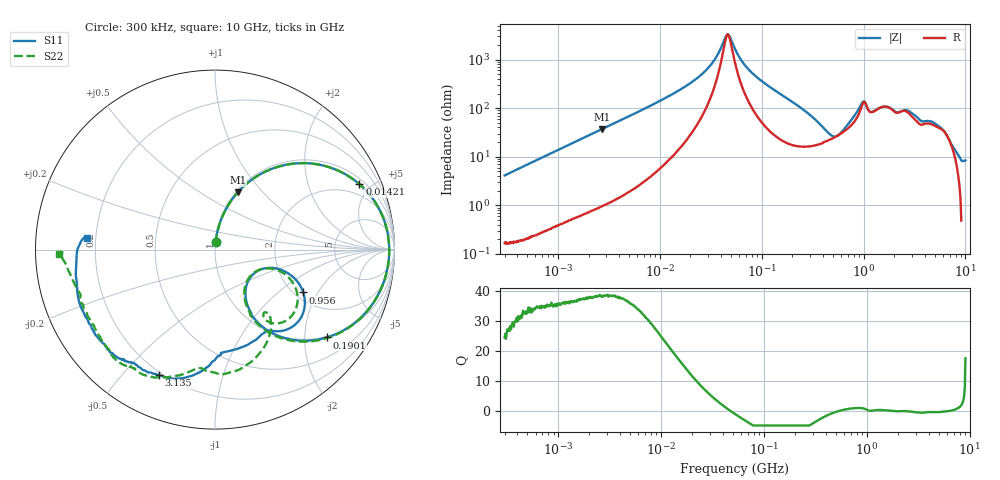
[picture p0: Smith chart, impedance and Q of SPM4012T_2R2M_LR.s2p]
! S-Parameter Data Generated by TDK Corporation
! Copyright(C) 2019 TDK Corporation.
! All Rights Reserved.
! TDK P/N: SPM4012T-2R2M-LR (Inductor)
! Property: L=2.2uH at 100kHz
! Size(LxWxT): 4.4x4.1x1.2mm
! Model Type: s2p (Touchstone File Format Version 1.0)
! Frequency: DC=Yes Start=0.3MHz Stop=10000MHz 802points Log-sweep
! Model Generated on Sep. 23, 2019
! Port Assignments:
!  1 ---@@@--- 2
! Applicable Conditions:
!  Temperature = 25 degC
!  DC Bias Current = 0 A
!  Small Signal Operation
! Terms and conditions regarding TDK Simulation Models
! (1)This simulation model is being provided solely for informational purposes. Please refer to the specifications of the products in terms of detailed characteristics of such products.
! (2)In no event shall TDK Corporation of any of its subsidiaries be liable for any loss or damage arising, directly or indirectly,
!  From any information contained in this simulation model, including, but not limited to loss or damages arising from any inaccuracies, omissions or errors in connection with such information.
! (3)Any and all copyrights on this simulation model are owned by TDK Corporation.
!  Duplication or redistribution of this simulation model without prior written permission from TDK Corporation is prohibited.
! (4)This simulation model is subject to any modification or change without any prior notice.
! (5)Neither TDK Corporation nor any of its subsidiaries shall make any warranty, express or implied,
!  Including but not limited to the correctness, implied warranties of merchantability and fitness for a particular purpose with respect to this simulation models.
! (6)The use of this simulation model shall be deemed to have consented to the terms and conditions hereof.
# Hz S MA R 50
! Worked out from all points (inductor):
!   801 points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, 300 kHz to 10 GHz, reference 50 ohm
!   read as one part in series: L = 2.19 uH near 318.3 kHz
!   highest Q = 38.6 at 2.728 MHz (marker M1), where L = 2.16 uH
!   self-resonance near 46.59 MHz
!   S11 on the Smith chart (normalised r, x): 300 kHz: 1.00, +0.08; 14.21 MHz: 1.28, +4.26; 190.1 MHz: 0.97, -2.56; 956 MHz: 2.22, -1.51; 3.135 GHz: 0.19, -0.63; 10 GHz: 0.16, +0.05
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300000  0.04018 85.3  0.9974 -2.4  0.9976 -2.4  0.03992 85.1
1713600  0.2257 75.4  0.9682 -13.1  0.9681 -13.1  0.2256 75.3
2728124  0.3438 68.3  0.93 -20.2  0.9302 -20.2  0.3438 68.3
9671944  0.7893 35.3  0.5838 -52.4  0.5839 -52.4  0.7892 35.3
1.421446e7  0.8835 24.4  0.4217 -62.4  0.4218 -62.4  0.8834 24.3
2.987769e7  0.9633 7.0  0.1435 -72.3  0.1436 -72.3  0.9633 6.9
4.564296e7  0.9706 -1.3  0.03004 -13.5  0.03006 -13.5  0.9706 -1.4
5.477226e7  0.9682 -4.9  0.05857 53.6  0.05859 53.6  0.9681 -5.0
8.622688e7  0.9462 -14.6  0.2016 65.6  0.2016 65.6  0.946 -14.8
1.900804e8  0.7923 -38.2  0.5233 44.7  0.5234 44.7  0.7914 -38.7
3.126428e8  0.5579 -55.9  0.7183 21.1  0.7184 21.1  0.5553 -56.8
4.448526e8  0.3494 -59.4  0.7798 1.1  0.7799 1.1  0.3443 -60.2
5.99416e8  0.2507 -38.0  0.7573 -17.5  0.7573 -17.5  0.2457 -37.6
7.956093e8  0.355 -17.1  0.6419 -36.8  0.6419 -36.8  0.3641 -18.2
9.560117e8  0.5467 -25.9  0.4462 -45.3  0.4463 -45.3  0.5404 -31.5
1.10164e9  0.5871 -50.5  0.4552 -28.5  0.4552 -28.6  0.4881 -54.1
1.307877e9  0.5388 -60.1  0.4671 -41.8  0.4672 -41.8  0.4797 -50.4
1.767019e9  0.5684 -80.1  0.3709 -44.9  0.371 -44.9  0.6627 -73.6
3.135132e9  0.7668 -114.2  0.2992 -57.1  0.2992 -57.2  0.789 -115.2
6.172341e9  0.8159 -141.5  0.2508 -86.9  0.2511 -87.1  0.7979 -144.9
7.875699e9  0.792 -166.3  0.2242 -109.0  0.2244 -109.1  0.8079 -167.1
1e10  0.7189 174.7  0.1687 -123.4  0.1687 -123.5  0.8669 -178.2
